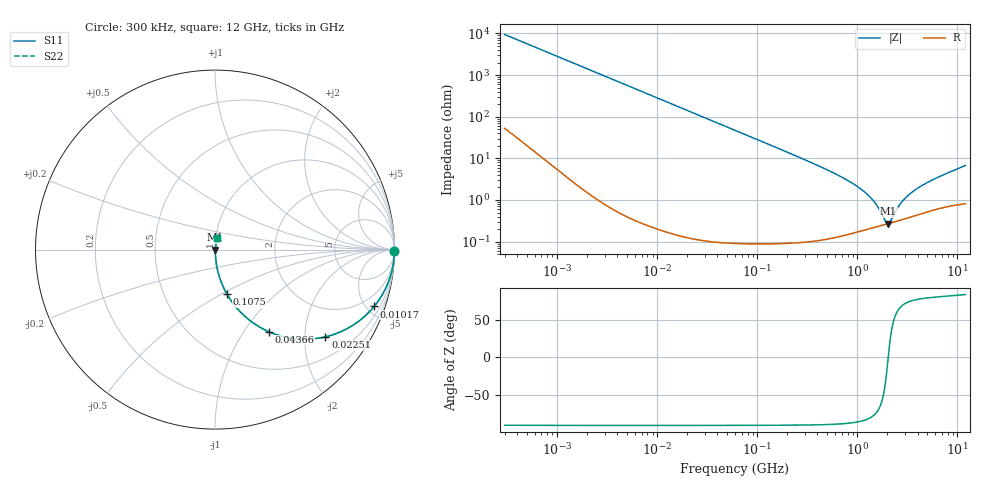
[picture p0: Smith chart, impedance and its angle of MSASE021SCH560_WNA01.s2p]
! MSASE021SCH560_WNA01  S-PARAMETER MODEL  ( Standard Model )
! Model Generated by TAIYO YUDEN Corporation (http://www.ty-top.com)
! Version 3.0
! TAIYO YUDEN Control No. 231201
! Copyright(c) 2016 TAIYO YUDEN CO.,LTD. All Rights Reserved.
! Product Description (link to TY-COMPAS)
! https://ds.yuden.co.jp/TYCOMPAS/or/detail?pn=MSASE021SCH560JWNA01&u=M
! Products Name : Multilayer Ceramic Capacitors
! Characteristics :
!  Capacitance : 56 [pF] , Rated Voltage : 16 [V] , TCC : CH / C0H
!  Case Size : 0.25 x 0.125 / 0.0098 x 0.0049 [mm/inch] , Thickness : 0.125 / 0.0049 [mm/inch]
!  (Conditions: Temperature = 25 [degC] , DC Bias Voltage = 0 [V])
! External Node Assignments :
!  1  o---| |---o  2
! GND o---------o GND
! Frequency Range : 0.3MHz  -  12000MHz  [ 401 STEP ]
# MHZ S RI R 50
! Freq[MHz].  S11 Real  S11 Imag  S21 Real  S21 Imag  S12 Real  S12 Imag  S22 Real  S22 Imag
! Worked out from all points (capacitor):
!   401 points, 300 kHz to 12 GHz, reference 50 ohm
!   read as one part in series: C = 56 pF near 316.3 kHz
!   lowest |Z| = 270 mohm at 2.034 GHz (marker M1)
!   series resonance near 2.034 GHz, so ESL is about 110 pH
!   S11 on the Smith chart (normalised r, x): 300 kHz: open; 10.17 MHz: 1.00, -5.60; 22.51 MHz: 1.00, -2.53; 43.66 MHz: 1.00, -1.30; 107.5 MHz: 1.00, -0.53; 12 GHz: 1.02, +0.13
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0.3  0.9998 -0.0106  0.00017 0.0106  0.00017 0.0106  0.9998 -0.0106
1.769972  0.9961 -0.0619  0.00392 0.0619  0.00392 0.0619  0.9961 -0.0619
4.473491  0.9758 -0.1533  0.0242 0.1533  0.0242 0.1533  0.9758 -0.1533
10.16966  0.8867 -0.3166  0.1133 0.3166  0.1133 0.3166  0.8867 -0.3166
10.44266  0.8813 -0.3231  0.1187 0.3231  0.1187 0.3231  0.8813 -0.3231
15.13155  0.7796 -0.4141  0.2204 0.4141  0.2204 0.4141  0.7796 -0.4141
22.51442  0.6152 -0.4861  0.3848 0.4861  0.3848 0.4861  0.6152 -0.4861
30.94016  0.4586 -0.4977  0.5414 0.4977  0.5414 0.4977  0.4586 -0.4977
43.66058  0.2985 -0.4569  0.7015 0.4569  0.7015 0.4569  0.2985 -0.4569
60  0.184 -0.3866  0.816 0.3866  0.816 0.3866  0.184 -0.3866
107.4644  0.0659 -0.2465  0.9341 0.2465  0.9341 0.2465  0.0659 -0.2465
353.9943  0.00699 -0.077  0.993 0.077  0.993 0.077  0.00699 -0.077
723.8279  0.00253 -0.0337  0.9975 0.0337  0.9975 0.0337  0.00253 -0.0337
1135.593  0.00212 -0.0167  0.9979 0.0167  0.9979 0.0167  0.00212 -0.0167
1480.043  0.00227 -0.00868  0.9977 0.00868  0.9977 0.00868  0.00227 -0.00868
1878.541  0.00256 -0.00212  0.9974 0.00212  0.9974 0.00212  0.00256 -0.00212
2033.931  0.00269 1.42e-07  0.9973 -1.42e-07  0.9973 -1.42e-07  0.00269 1.42e-07
2088.533  0.00274 0.000701  0.9973 -0.000701  0.9973 -0.000701  0.00274 0.000701
2722.03  0.00335 0.00771  0.9966 -0.00771  0.9966 -0.00771  0.00335 0.00771
3642.919  0.00433 0.0158  0.9957 -0.0158  0.9957 -0.0158  0.00433 0.0158
5715.274  0.00657 0.0301  0.9934 -0.0301  0.9934 -0.0301  0.00657 0.0301
12000  0.0124 0.0654  0.9876 -0.0654  0.9876 -0.0654  0.0124 0.0654
